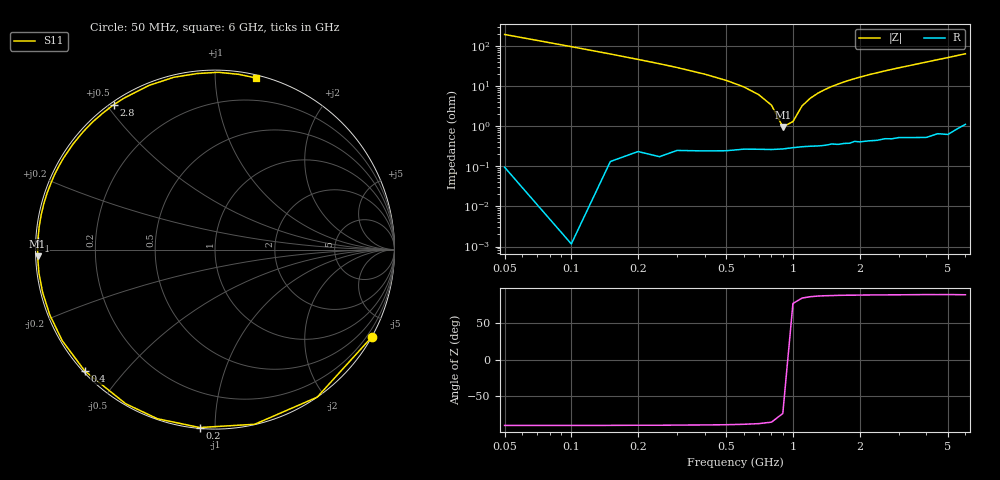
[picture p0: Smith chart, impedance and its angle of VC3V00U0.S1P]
! Infineon Technologies  Discrete & RF Semiconductors
! BBY 56-03
! Si Tuning Diode in SOD323
! VR = 3 V
! S-Parameters:  June  1999
# GHz  S  MA  R  50
!  f  S11
! GHz  MAG  ANG
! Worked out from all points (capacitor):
!   34 points, 50 MHz to 6 GHz, reference 50 ohm
!   read as one part to ground: C = 16.5 pF near 50 MHz
!   lowest |Z| = 955 mohm at 900 MHz (marker M1)
!   series resonance near 942 MHz, so ESL is about 1.7 nH
!   S11 on the Smith chart (normalised r, x): 50 MHz: 0.00, -3.84; 200 MHz: 0.00, -0.92; 400 MHz: 0.00, -0.39; 1 GHz: 0.01, +0.03; 2.8 GHz: 0.01, +0.52; 6 GHz: 0.02, +1.27
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0.05  0.9998 -29.2
0.1  1 -55.3
0.15  0.998 -77.2
0.2  0.995 -94.9
0.25  0.9954 -108.8
0.3  0.9926 -120.1
0.4  0.9917 -137.0
0.5  0.991 -149.2
0.6  0.9898 -158.5
0.7  0.9896 -166.1
0.8  0.9897 -172.4
0.9  0.9893 -177.9
1  0.9885 177.1
1.2  0.9876 168.6
1.3  0.9875 164.8
1.6  0.9868 154.8
1.8  0.9862 148.8
2  0.9855 143.4
2.2  0.9851 138.3
2.4  0.9851 133.7
2.8  0.9849 125.0
3  0.9844 121.0
3.5  0.9859 111.9
4  0.9872 103.4
4.5  0.9859 95.7
5  0.9879 88.9
5.5  0.9854 82.3
6  0.9832 76.5
